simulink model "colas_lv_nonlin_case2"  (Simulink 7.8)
settings: Solver=ode15s  SolverMode=SingleTasking  StartTime=0  StopTime=130  MaxStep=1  RelTol=1e-5  AbsTol=1e-5

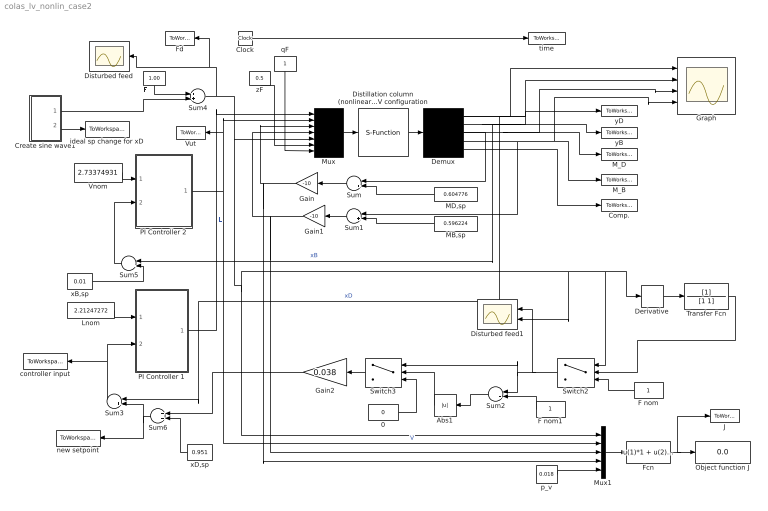
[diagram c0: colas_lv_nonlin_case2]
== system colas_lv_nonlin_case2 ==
  0 : Constant  Value=0
  Abs1 : Abs
  Clock : Clock
  Comp. : ToWorkspace  VariableName=Comp  SaveFormat=Structure With Time
  Create sine wave1 : Subsystem
  Demux : Demux  Outputs=[1,1,1,1,82]
  Derivative : Derivative
  Distillation column (nonlinear)  LV configuration : S-Function  FunctionName=scolas_orig  EnableBusSupport=off
  Disturbed feed : Scope
  Disturbed feed1 : Scope  NumInputPorts=2
  F : Constant  Value=1.00
  F nom : Constant
  F nom1 : Constant
  Fcn : Fcn  Expr=u(1)*1 + u(2)*u(5) - u(3)*1-u(4)*2
  Fd : ToWorkspace  VariableName=Fd  SaveFormat=Structure With Time
  Gain : Gain  Gain=-10
  Gain1 : Gain  Gain=-10
  Gain2 : Gain  Gain=0.038
  Graph : Scope  NumInputPorts=4
  J : ToWorkspace  VariableName=J  SaveFormat=Structure With Time
  Lnom : Constant  Value=2.21247272
  MB,sp : Constant  Value=0.596224
  MD,sp : Constant  Value=0.604776
  M_B : ToWorkspace  VariableName=y4  SaveFormat=Structure With Time
  M_D : ToWorkspace  VariableName=y3  SaveFormat=Structure With Time
  Mux : Mux  Inputs=7
  Mux1 : Mux  Inputs=5
  Object function J : Display
  PI Controller 1 : Subsystem
  PI Controller 2 : Subsystem
  Sum{,1..3,5} (5 alike) : Sum  Inputs=-+
  Sum4 : Sum
  Sum6 : Sum
  Switch2 : Switch  Criteria=u2 ~= 0
  Switch3 : Switch  Criteria=u2 > Threshold  Threshold=0.29
  Transfer Fcn : TransferFcn  Denominator=[1 1]
  Vnom : Constant  Value=2.73374931
  Vut : ToWorkspace  VariableName=Vut  SaveFormat=Structure With Time
  controller input : ToWorkspace  VariableName=inp  SaveFormat=Structure With Time
  ideal sp change for xD : ToWorkspace  VariableName=idealsp  SaveFormat=Structure With Time
  new setpoint : ToWorkspace  VariableName=setp  SaveFormat=Structure With Time
  p_v : Constant  Value=0.018
  qF : Constant
  time : ToWorkspace  VariableName=t  SaveFormat=Array
  xB,sp : Constant  Value=0.01
  xD,sp : Constant  Value=0.951
  yB : ToWorkspace  VariableName=y2  SaveFormat=Structure With Time
  yD : ToWorkspace  VariableName=y1  SaveFormat=Structure With Time
  zF : Constant  Value=0.5
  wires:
  qF/1 -> Mux/7
  Demux/1 -> Graph/1, yD/1, Sum3/1  "xD"
  Gain1/1 -> Mux/4, Mux1/3
  Sum1/1 -> Gain1/1
  MB,sp/1 -> Sum1/2
  Demux/4 -> Sum1/1, M_B/1, Graph/4
  Demux/3 -> Sum/1, Graph/3, M_D/1
  Gain/1 -> Mux/3, Mux1/4
  MD,sp/1 -> Sum/2
  Sum/1 -> Gain/1
  Mux/1 -> Distillation column (nonlinear)  LV configuration/1
  Distillation column (nonlinear)  LV configuration/1 -> Demux/1
  Clock/1 -> time/1
  zF/1 -> Mux/6
  Demux/5 -> Comp./1
  Sum3/1 -> PI Controller 1/2(SP error), controller input/1
  Sum5/1 -> PI Controller 2/2(SP error)
  Sum4/1 -> Disturbed feed/1, Fd/1, Mux/5, Mux1/1, Derivative/1, Switch2/1, Disturbed feed1/2
  p_v/1 -> Mux1/5
  Fcn/1 -> Object function J/1, J/1
  Mux1/1 -> Fcn/1
  Lnom/1 -> PI Controller 1/1(Nom. value)
  PI Controller 1/1(L) -> Mux/1  "L"
  Vnom/1 -> PI Controller 2/1(Nom. value)
  PI Controller 2/1(V) -> Mux1/2, Mux/2, Vut/1  "V"
  xB,sp/1 -> Sum5/2
  F nom/1 -> Switch2/3
  F/1 -> Sum4/1
  xD,sp/1 -> Sum6/2
  Demux/2 -> Sum5/1, yB/1, Graph/2  "xB"
  Derivative/1 -> Transfer Fcn/1
  Transfer Fcn/1 -> Switch2/2
  Switch2/1 -> Sum2/1, Switch3/1, Disturbed feed1/1
  F nom1/1 -> Sum2/2
  Sum2/1 -> Abs1/1
  Switch3/1 -> Gain2/1
  Abs1/1 -> Switch3/2
  0/1 -> Switch3/3
  Create sine wave1/1(Out1) -> Sum4/2
  Gain2/1 -> Sum6/1
  Create sine wave1/2(Out2) -> ideal sp change for xD/1
  Sum6/1 -> new setpoint/1, Sum3/2

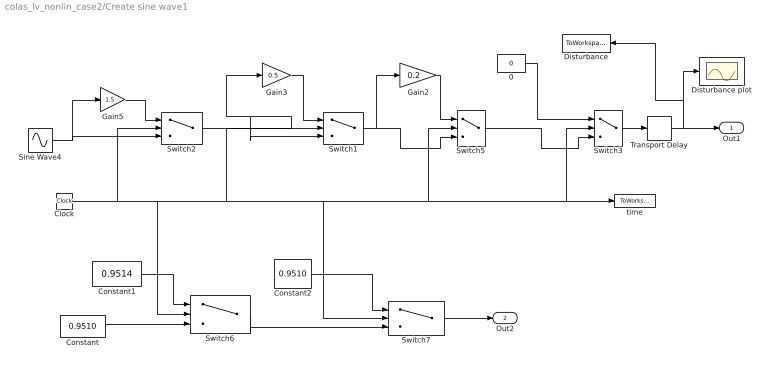
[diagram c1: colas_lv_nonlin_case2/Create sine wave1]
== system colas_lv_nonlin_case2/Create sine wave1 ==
  0 : Constant  Value=0
  Clock : Clock
  Constant : Constant  Value=0.9510
  Constant1 : Constant  Value=0.9514
  Constant2 : Constant  Value=0.9510
  Disturbance : ToWorkspace  VariableName=wa  SaveFormat=Structure With Time
  Disturbance plot : Scope
  Gain2 : Gain  Gain=0.2
  Gain3 : Gain  Gain=0.5
  Gain5 : Gain  Gain=1.5
  Sine Wave4 : Sin  Amplitude=0.2  SampleTime=0
  Switch1 : Switch  Criteria=u2 > Threshold  Threshold=62.9
  Switch2 : Switch  Criteria=u2 > Threshold  Threshold=28.3
  Switch3 : Switch  Criteria=u2 > Threshold  Threshold=106.8
  Switch5 : Switch  Criteria=u2 > Threshold  Threshold=87
  Switch6 : Switch  Criteria=u2 > Threshold  Threshold=38.3
  Switch7 : Switch  Criteria=u2 > Threshold  Threshold=72.9
  Transport Delay : TransportDelay  DelayTime=10
  time : ToWorkspace  VariableName=t1  SaveFormat=Array
  Out1 : Outport
  Out2 : Outport  Port=2
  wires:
  Clock/1 -> Switch2/2, Switch1/2, time/1, Switch3/2, Switch5/2, Switch7/2, Switch6/2
  Switch2/1 -> Gain3/1, Switch1/3
  Gain5/1 -> Switch2/1
  Gain3/1 -> Switch1/1
  Sine Wave4/1 -> Switch2/3, Gain5/1
  0/1 -> Switch3/1
  Transport Delay/1 -> Out1/1, Disturbance plot/1, Disturbance/1
  Switch3/1 -> Transport Delay/1
  Switch1/1 -> Switch5/3, Gain2/1
  Switch5/1 -> Switch3/3
  Gain2/1 -> Switch5/1
  Constant/1 -> Switch6/3
  Constant1/1 -> Switch6/1
  Switch6/1 -> Switch7/3
  Constant2/1 -> Switch7/1
  Switch7/1 -> Out2/1

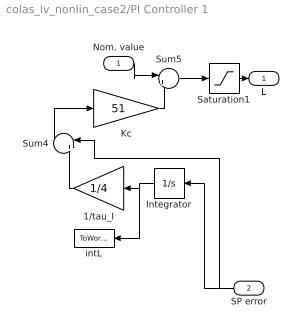
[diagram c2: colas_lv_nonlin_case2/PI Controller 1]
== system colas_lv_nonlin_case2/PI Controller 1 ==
  Nom. value : Inport
  SP error : Inport  Port=2
  1/tau_I : Gain  Gain=1/4
  Integrator : Integrator  InitialCondition=0.0004
  Kc : Gain  Gain=51
  Saturation1 : Saturate  UpperLimit=inf  LowerLimit=0
  Sum4 : Sum  Inputs=|++
  Sum5 : Sum  Inputs=|++
  intL : ToWorkspace  VariableName=intL  SaveFormat=Array
  L : Outport
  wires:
  SP error/1 -> Sum4/1, Integrator/1
  Integrator/1 -> 1/tau_I/1, intL/1
  1/tau_I/1 -> Sum4/2
  Sum4/1 -> Kc/1
  Kc/1 -> Sum5/2
  Nom. value/1 -> Sum5/1
  Saturation1/1 -> L/1
  Sum5/1 -> Saturation1/1

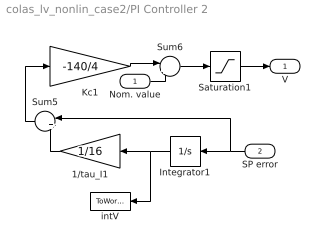
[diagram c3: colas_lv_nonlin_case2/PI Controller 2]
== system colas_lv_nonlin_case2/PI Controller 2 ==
  Nom. value : Inport
  SP error : Inport  Port=2
  1/tau_I1 : Gain  Gain=1/16
  Integrator1 : Integrator  InitialCondition=-0.0002
  Kc1 : Gain  Gain=-140/4
  Saturation1 : Saturate  UpperLimit=inf  LowerLimit=0
  Sum5 : Sum  Inputs=|++
  Sum6 : Sum  Inputs=|++
  intV : ToWorkspace  VariableName=intV  SaveFormat=Array
  V : Outport
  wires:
  SP error/1 -> Sum5/1, Integrator1/1
  Integrator1/1 -> 1/tau_I1/1, intV/1
  1/tau_I1/1 -> Sum5/2
  Sum5/1 -> Kc1/1
  Kc1/1 -> Sum6/1
  Nom. value/1 -> Sum6/2
  Sum6/1 -> Saturation1/1
  Saturation1/1 -> V/1
